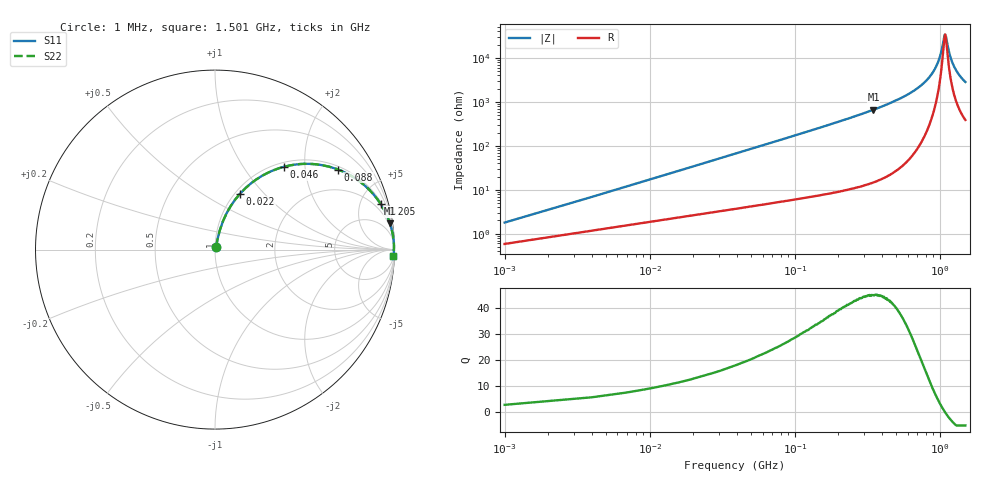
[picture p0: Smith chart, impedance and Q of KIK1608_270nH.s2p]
!version-2
!date-01.2022
!Series
# MHz S RI R 50
!Freq ReS11 ImS11 ReS21 ImS21 ReS12 ImS12 ReS22 ImS22
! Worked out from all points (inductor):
!   501 points, 1 MHz to 1.501 GHz, reference 50 ohm
!   read as one part in series: L = 270 nH near 7 MHz
!   highest Q = 44.9 at 349 MHz (marker M1), where L = 301 nH
!   self-resonance near 1.087 GHz
!   S11 on the Smith chart (normalised r, x): 1 MHz: 1.01, +0.03; 22 MHz: 1.06, +0.75; 46 MHz: 1.08, +1.56; 88 MHz: 1.11, +3.01; 205 MHz: 1.18, +7.21; 1.501 GHz: 9, -56
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1  0.00612 0.0168  0.9939 -0.0168  0.9939 -0.0168  0.00612 0.0168
10  0.0447 0.1591  0.9553 -0.1591  0.9553 -0.1591  0.0447 0.1591
16  0.0872 0.2421  0.9128 -0.2421  0.9128 -0.2421  0.0872 0.2421
22  0.1403 0.3124  0.8597 -0.3124  0.8597 -0.3124  0.1403 0.3124
31  0.2314 0.3917  0.7686 -0.3917  0.7686 -0.3917  0.2314 0.3917
46  0.3856 0.4618  0.6144 -0.4618  0.6144 -0.4618  0.3856 0.4618
67  0.5633 0.4752  0.4367 -0.4752  0.4367 -0.4752  0.5633 0.4752
88  0.687 0.4455  0.313 -0.4455  0.313 -0.4455  0.687 0.4455
136  0.8387 0.353  0.1613 -0.353  0.1613 -0.353  0.8387 0.353
205  0.9231 0.2541  0.0769 -0.2541  0.0769 -0.2541  0.9231 0.2541
253  0.9492 0.208  0.0508 -0.208  0.0508 -0.208  0.9492 0.208
349  0.9744 0.1471  0.0256 -0.1471  0.0256 -0.1471  0.9744 0.1471
502  0.9893 0.0912  0.0107 -0.0912  0.0107 -0.0912  0.9893 0.0912
751  0.9962 0.0409  0.0038 -0.0409  0.0038 -0.0409  0.9962 0.0409
904  0.9972 0.0201  0.00279 -0.0201  0.00279 -0.0201  0.9972 0.0201
1003  0.9973 0.00885  0.00273 -0.00885  0.00273 -0.00885  0.9973 0.00885
1075  0.9971 0.00139  0.00289 -0.00139  0.00289 -0.00139  0.9971 0.00139
1090  0.9971 -9.73e-05  0.00294 9.73e-05  0.00294 9.73e-05  0.9971 -9.73e-05
1171  0.9967 -0.00779  0.00331 0.00779  0.00331 0.00779  0.9967 -0.00779
1252  0.9962 -0.015  0.00381 0.015  0.00381 0.015  0.9962 -0.015
1360  0.9953 -0.024  0.00467 0.024  0.00467 0.024  0.9953 -0.024
1501  0.994 -0.0347  0.00605 0.0347  0.00605 0.0347  0.994 -0.0347
